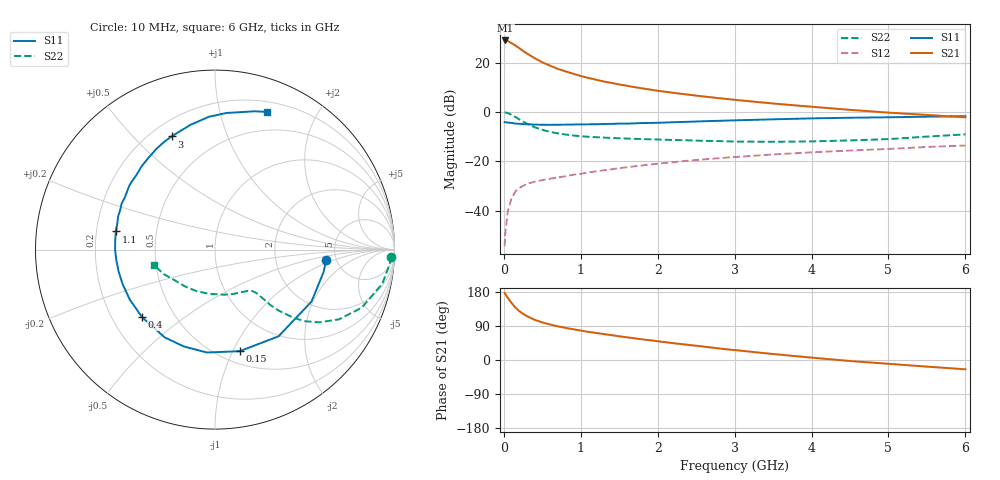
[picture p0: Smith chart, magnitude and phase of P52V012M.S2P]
! SIEMENS Small Signal Semiconductors
! BFP183
! Si NPN RF Bipolar Junction Transistor in SOT143
! VCE = 2 V  IC = 12 mA
! Common Emitter S-Parameters:  March  1996
# GHz  S  MA  R  50
!  f  S11  S21  S12  S22
! GHz  MAG  ANG  MAG  ANG  MAG  ANG  MAG  ANG
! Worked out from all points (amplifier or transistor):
!   36 points, 10 MHz to 6 GHz, reference 50 ohm
!   highest |S21| = 29.0 dB at 20 MHz (marker M1)
!   |S21| within 3 dB of that: start of sweep to 195 MHz
!   unconditionally stable (mu >= 1): 997.3 MHz to 5.536 GHz
!   at 250 MHz: K = 0.37, MSG = 27.4 dB, |S12| = -30.0 dB
!   at 1.4 GHz: K = 1.12, MAG = 15.4 dB, |S12| = -23.2 dB
!   at 6 GHz: K = 0.95, MSG = 5.7 dB, |S12| = -13.6 dB
!   S11 on the Smith chart (normalised r, x): 10 MHz: 4.12, -0.80; 150 MHz: 0.62, -1.06; 400 MHz: 0.33, -0.36; 1.1 GHz: 0.28, +0.08; 3 GHz: 0.28, +0.65; 6 GHz: 0.30, +1.40
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0.01  0.6215 -5.5  27.98 176.9  0.0019 85.0  0.9799 -2.3
0.02  0.6179 -11.6  28.17 173.9  0.0036 79.0  0.9765 -4.7
0.05  0.6108 -28.3  27.45 164.3  0.0095 78.5  0.9517 -11.5
0.1  0.5989 -53.8  24.93 150.5  0.0177 67.1  0.8792 -21.6
0.15  0.5824 -76.3  22.33 138.6  0.0244 59.0  0.7919 -29.4
0.2  0.5751 -94.5  19.7 129.1  0.0287 53.7  0.7085 -34.9
0.25  0.5669 -107.9  17.27 121.7  0.0317 49.5  0.6376 -38.7
0.3  0.5639 -119.8  15.36 115.8  0.035 47.5  0.5777 -41.0
0.4  0.5539 -137.1  12.33 106.1  0.0385 44.2  0.4905 -43.8
0.5  0.5505 -149.5  10.15 99.2  0.0414 42.9  0.4339 -45.1
0.6  0.5495 -159.3  8.694 93.7  0.0443 43.0  0.3952 -45.4
0.7  0.5509 -167.5  7.492 89.0  0.047 43.6  0.3681 -45.8
0.9  0.5567 -179.8  5.964 81.3  0.0533 44.6  0.3342 -46.4
1.1  0.5619 169.6  4.908 74.2  0.0594 45.7  0.314 -47.8
1.5  0.5802 153.9  3.614 62.5  0.0724 46.2  0.2927 -52.0
1.8  0.5961 143.1  3.009 54.5  0.0823 46.0  0.2812 -56.8
2.2  0.6188 131.3  2.447 44.5  0.0959 44.3  0.2703 -64.4
3  0.6756 111.0  1.763 26.2  0.122 39.3  0.2512 -83.9
3.5  0.7089 101.0  1.483 15.8  0.1374 35.8  0.2484 -98.1
4.5  0.7636 85.3  1.104 -2.7  0.165 27.8  0.2648 -129.3
5.5  0.8017 74.0  0.87 -17.5  0.1951 20.5  0.3166 -154.6
6  0.82 69.3  0.779 -24.5  0.2086 16.0  0.3513 -165.7
